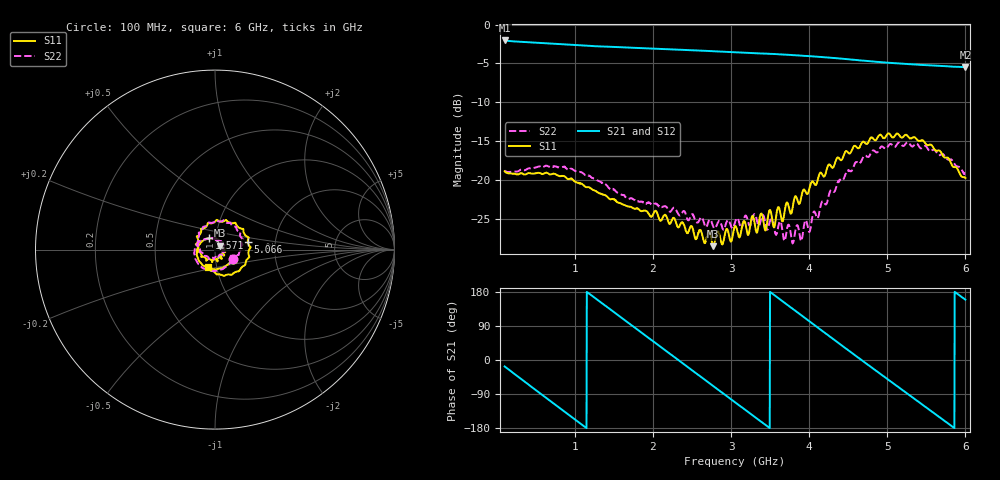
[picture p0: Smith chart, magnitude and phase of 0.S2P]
!Agilent Technologies,E5071C,MY46316741,A.11.02
!Date: Thu Dec 16 09:44:59 2021
!Data & Calibration Information:
!Freq	S11:SOLT4(ON)	S21:SOLT4(ON)	S12:SOLT4(ON)	S22:SOLT4(ON)
!PortZ  Port1:50+j0  Port2:50+j0
!Above PortZ is port z conversion or system Z0 setting when saving the data.
!When reading, reference impedance value at option line is always used.
# Hz S dB R 50
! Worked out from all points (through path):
!   1593 points, 100 MHz to 6 GHz, reference 50 ohm
!   highest |S21| = -2.04 dB at 100 MHz (marker M1); lowest = -5.5 dB at 6 GHz (marker M2)
!   group delay of S21, straight-line fit = 426 ps
!   lowest |S11| = -28.5 dB at 2.772 GHz (marker M3), VSWR 1.08, Z = 53 + j2.42 ohm
!   |S11| at or under -10 dB: start of sweep to end of sweep
!   |S22| runs from -28.2 to -15.1 dB; largest |S21 - S12| = 0.0049
!   S11 on the Smith chart (normalised r, x): 100 MHz: 1.22, -0.13; 1.571 GHz: 0.93, +0.12; 5.066 GHz: 1.44, +0.13; 6 GHz: 0.91, -0.18
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1e8  -18.89 -27.3  -2.04 -17.0  -2.05 -17.0  -18.78 -26.8
3.594221e8  -19.32 -78.1  -2.25 -57.6  -2.26 -57.6  -18.76 -76.5
5.780779e8  -19.24 -118.4  -2.39 -91.7  -2.40 -91.6  -18.35 -115.1
8.041457e8  -19.52 -155.5  -2.52 -126.7  -2.53 -126.6  -18.38 -149.9
1.085804e9  -20.49 165.9  -2.68 -170.1  -2.69 -170.1  -19.03 175.1
1.319284e9  -21.73 140.2  -2.81 154.1  -2.82 154.1  -20.20 152.8
1.571294e9  -22.97 118.3  -2.90 115.4  -2.91 115.5  -21.81 134.3
1.80848e9  -23.70 101.8  -3.01 79.0  -3.02 79.0  -22.76 122.9
2.067902e9  -24.68 86.8  -3.12 39.3  -3.12 39.4  -23.28 110.4
2.405151e9  -26.05 61.0  -3.25 -12.5  -3.27 -12.5  -24.08 92.3
2.772048e9  -28.54 37.5  -3.42 -68.8  -3.44 -68.7  -26.03 79.7
3.05e9  -25.99 14.9  -3.56 -111.4  -3.58 -111.3  -25.50 60.7
3.528078e9  -25.20 -53.0  -3.78 175.2  -3.78 175.4  -25.15 9.1
3.791206e9  -23.38 -126.4  -3.93 134.6  -3.93 134.8  -28.10 -51.4
4.035804e9  -20.21 -173.9  -4.08 97.0  -4.09 97.2  -25.02 -123.4
4.27299e9  -18.15 143.0  -4.27 60.5  -4.27 60.7  -21.36 -171.7
4.550942e9  -16.06 89.1  -4.51 18.0  -4.51 18.2  -18.71 140.2
5.017902e9  -14.00 19.7  -4.91 -52.8  -4.92 -52.5  -15.56 74.8
5.06608e9  -14.54 13.1  -4.95 -60.0  -4.96 -59.7  -15.55 72.1
5.444095e9  -14.93 -41.2  -5.19 -117.0  -5.19 -116.7  -15.89 25.1
5.72946e9  -17.10 -80.1  -5.35 -160.1  -5.33 -159.7  -16.85 -2.1
6e9  -19.76 -112.1  -5.47 159.2  -5.46 159.5  -19.22 -26.3
